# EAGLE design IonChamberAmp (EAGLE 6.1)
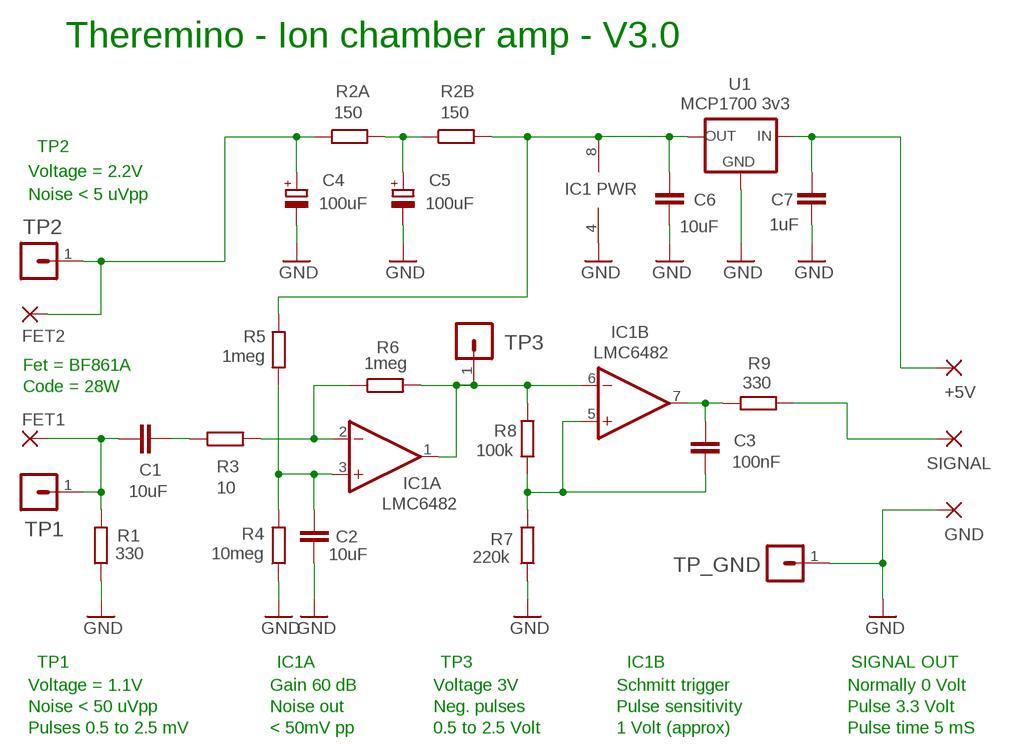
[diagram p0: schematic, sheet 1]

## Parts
+5V  WIREPAD1,6/0,8  [1,6/0,8]
C1  10uF  C-EUC0805  [C0805]
C2  10uF  C-EUC0805  [C0805]
C3  100nF  C-EUC0805  [C0805]
C4  100uF  CPOL-EUE2-5B  [E2-5B]
C5  100uF  CPOL-EUE2-5B  [E2-5B]
C6  10uF  C-EUC0805  [C0805]
C7  1uF  C-EUC0805  [C0805]
FET1  WIREPADSMD1,90-2,54  [SMD1,90-2,54]
FET2  WIREPADSMD1,90-2,54  [SMD1,90-2,54]
GND  WIREPAD1,6/0,8  [1,6/0,8]
IC1  LMC6482  TL072P  [DIL08]
R1  330  R-EU_R0805  [R0805]
R2A  150  R-EU_R0805  [R0805]
R2B  150  R-EU_R0805  [R0805]
R3  10  R-EU_R0805  [R0805]
R4  10meg  R-EU_R0805  [R0805]
R5  1meg  R-EU_R1206_L  [R1206_L]
R6  1meg  R-EU_R0805  [R0805]
R7  220k  R-EU_R0805  [R0805]
R8  100k  R-EU_R0805  [R0805]
R9  330  R-EU_R0805  [R0805]
SIGNAL  WIREPAD1,6/0,8  [1,6/0,8]
TP1  MA01-1  [MA01-1]
TP2  MA01-1  [MA01-1]
TP3  MA01-1  [MA01-1]
TP_GND  MA01-1  [MA01-1]
U1  MCP1700 3v3  MCP1700SOT23L  [SOT23_L]

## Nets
GND: C2.1 C4.- C5.- C6.2 C7.2 GND.1(P) IC1.4(P:V-) R1.1 R4.1 R7.1 TP_GND.1 U1.1(GND)
N$1: C3.2 IC1.5(B:+IN) R7.2 R8.1
N$2: C2.2 IC1.3(A:+IN) R4.2 R5.1
N$3: IC1.1(A:OUT) IC1.6(B:-IN) R6.2 R8.2 TP3.1
N$4: IC1.2(A:-IN) R3.2 R6.1
N$5: C3.1 IC1.7(B:OUT) R9.1
N$6: C1.2 FET1.1(P) R1.2 TP1.1
N$7: R9.2 SIGNAL.1(P)
N$8: +5V.1(P) C7.1 U1.3(IN)
N$10: C6.1 IC1.8(P:V+) R2B.2 R5.2 U1.2(OUT)
N$11: C1.1 R3.1
N$12: C5.+ R2A.2 R2B.1
TP2: C4.+ FET2.1(P) R2A.1 TP2.1

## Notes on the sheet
- Theremino - Ion chamber amp - V3.0
- TP2
- Voltage = 2.2V
- IC1 PWR
- Noise < 5 uVpp
- Fet = BF861A
- Code = 28W
- TP1 | IC1A | TP3 | IC1B | SIGNAL OUT
- Voltage = 1.1V | Gain 60 dB | Voltage 3V | Schmitt trigger | Normally 0 Volt
- Noise < 50 uVpp | Noise out | Neg. pulses | Pulse sensitivity | Pulse 3.3 Volt
- Pulses 0.5 to 2.5 mV | < 50mV pp | 0.5 to 2.5 Volt | 1 Volt (approx) | Pulse time 5 mS

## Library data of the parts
+5V FET1 FET2 GND SIGNAL = 00-LIVIO:WIREPAD: Wire PAD connect wire on PCB
C1-C3 C6 C7 = 00-LIVIO:C-EU: CAPACITOR, European symbol
C4 C5 = 00-LIVIO:CPOL-EU: POLARIZED CAPACITOR, European symbol
IC1 = linear:TL072: OP AMP
R1 R2A R2B R3-R9 = 00-LIVIO:R-EU_: RESISTOR, European symbol
TP1-TP3 TP_GND = 03-con-lstb-M:MA01-1: PIN HEADER
U1 = 00-LIVIO:MCP1700: Linear regulator Quescient courrent 1.8uA Input 2.3v to 6v Output 1.2v 1.8v 2.5v 3.0v 3.3v 5.0v

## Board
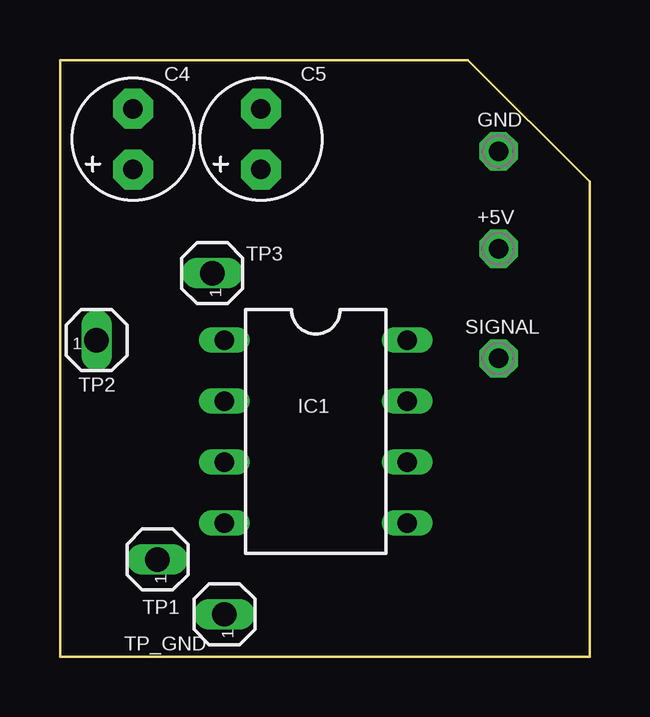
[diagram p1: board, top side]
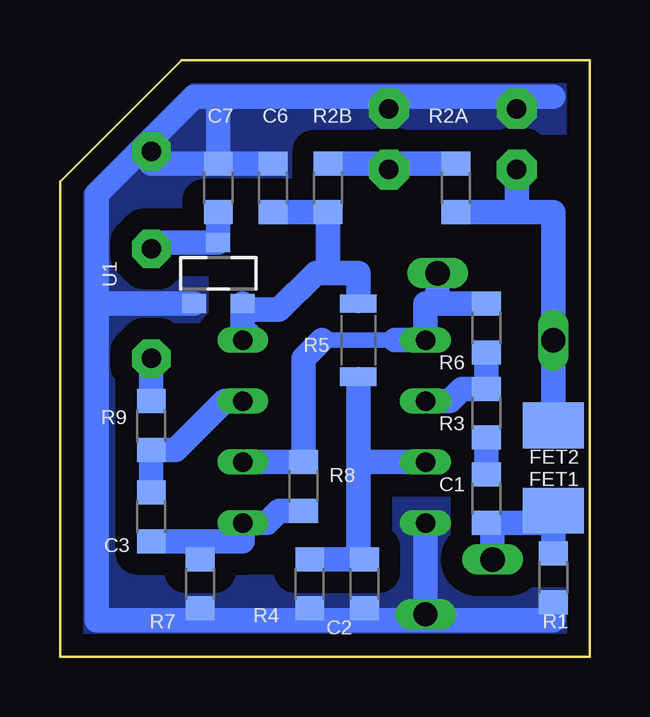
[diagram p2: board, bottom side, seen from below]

Size 22.1 x 24.89 mm. Coordinates in mm from the lower left corner, seen from the top.
Outline: 0,0 22.1,0 22.1,19.81 17.02,24.89 0,24.89 0,0
Copper layers (1*16): Top 0.035mm / dielectric 1.5mm / Bottom 0.035mm
Design rules: minimum track width 10mil, minimum drill 31mil, track to track 31mil, track to pad 31mil, pad to pad 31mil, via to via 31mil, smd to smd 31mil, copper to edge 31mil, drill to drill 8mil, minimum pad ring 5mil, minimum via ring 8mil, stop-mask expansion 4mil, vias tented up to drill 0mil, thermal gap 47mil

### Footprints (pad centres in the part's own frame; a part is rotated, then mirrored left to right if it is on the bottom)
1,6/0,8 = drill 0.813 pad 1.6 octagon: 1 0,0
C0805 = smd 1 x 1.2: 1 -1.016,0; 2 1.016,0
E2-5B = drill 0.813 pad 1.676 octagon: + -1.27,0; - 1.27,0
SMD1,90-2,54 = smd 1.905 x 2.54: 1 0,0
DIL08 = drill 0.813 long: 1 -3.81,-3.81; 2 -1.27,-3.81; 3 1.27,-3.81; 4 3.81,-3.81; 5 3.81,3.81; 6 1.27,3.81; 7 -1.27,3.81; 8 -3.81,3.81
R0805 = smd 1 x 1.2: 1 -1.016,0; 2 1.016,0
R1206_L = smd 0.762 x 1.524: 1 -1.524,0; 2 1.524,0
MA01-1 = drill 1.016 long: 1 0,0
SOT23_L = smd 1 x 0.8: 1 -1.016,-1.27; 2 1.016,-1.27; 3 0,1.27

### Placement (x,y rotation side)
+5V  18.29,17.02 0 top
C1  4.32,6.6 270 bottom
C2  9.4,3.05 90 bottom
C3  18.29,5.84 270 bottom
C4  3.05,21.59 90 top
C5  8.38,21.59 90 top
C6  13.21,19.56 90 bottom
C7  15.49,19.56 90 bottom
FET1  1.52,6.1 90 bottom
FET2  1.52,9.65 270 bottom
GND  18.29,21.08 0 top
IC1  10.67,9.4 270 top
R1  1.52,3.3 90 bottom
R2A  5.59,19.56 90 bottom
R2B  10.92,19.56 270 bottom
R3  4.32,10.16 90 bottom
R4  11.68,3.05 90 bottom
R5  9.65,13.21 90 bottom
R6  4.32,13.72 90 bottom
R7  16.26,3.05 90 bottom
R8  11.94,7.11 90 bottom
R9  18.29,9.65 90 bottom
SIGNAL  18.29,12.45 0 top
TP1  4.06,4.06 90 top
TP2  1.52,13.21 0 top
TP3  6.35,16 90 top
TP_GND  6.86,1.78 90 top
U1  15.49,16 0 bottom

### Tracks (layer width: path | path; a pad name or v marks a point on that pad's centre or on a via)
GND
  Bottom 1.016: 6.86,1.52 1.52,1.52 R1.1 | 6.86,1.52 9.4,1.52 | 9.4,1.52 11.68,1.52 | 11.68,1.52 R4.1 11.68,1.52 | 11.68,1.52 9.4,1.52 | 9.4,1.52 6.86,1.52 | 6.86,1.52 IC1.4 6.86,1.52 | 20.57,14.73 20.57,1.52 | 11.68,1.52 16.26,1.52 | 16.26,1.52 20.57,1.52 | 20.57,14.73 20.57,1.52 | 20.57,1.52 20.57,14.73 | 20.57,14.73 20.57,1.52 | 11.68,1.52 9.4,1.52 | 9.4,1.52 6.86,1.52 | 8.38,23.37 3.56,23.37 | 3.56,23.37 1.52,23.37 | C2.1 9.4,1.52 | U1.1 17.02,14.73 20.57,14.73 | C6.2 C7.2 | R7.1 16.26,1.52 | 3.56,23.37 C4.- | C5.- 8.38,23.37 | 8.38,23.37 15.49,23.37 | 15.49,23.37 16.51,23.37 20.57,19.3 20.57,14.73 | C7.2 15.49,23.37 | GND.1 18.29,20.57 C7.2
  pour Bottom (isolate 0.9, rank 6, no thermals): -1,-1 23.1,-1 23.1,25.89 -1,25.89
N$1
  Bottom 1.016: R8.1 12.95,6.1 13.46,5.59 IC1.5 14.48,4.83 16.26,4.83 | 16.26,4.83 R7.2 16.26,4.83 | 16.26,4.83 C3.2
N$2
  Bottom 0.813: 9.65,11.43 R5.1
  Bottom 1.016: R4.2 9.65,4.06 | 9.65,4.06 C2.2 9.65,4.06 | 9.65,4.06 9.65,8.13 | IC1.3 9.65,8.13 | 9.65,8.13 9.65,11.43
N$3
  Bottom 0.65: 8.13,13.21 11.18,13.21
  Bottom 1.016: 6.35,14.73 6.86,14.73 IC1.1 8.13,13.21 | 6.35,14.73 R6.2 | 11.18,13.21 11.94,12.45 R8.2 | R8.2 13.46,8.13 | 13.46,8.13 IC1.6 13.46,8.13 | 13.46,8.13 R8.2 | 6.35,14.73 TP3.1
N$4
  Bottom 1.016: IC1.2 5.84,10.67 5.33,11.18 R3.2 R6.1
N$5
  Bottom 1.016: C3.1 R9.1 17.27,8.64 15.24,10.67 IC1.7
N$6
  Bottom 1.016: 1.52,5.59 4.06,5.59 | 4.06,5.59 C1.2 | 1.52,5.59 FET1.1 | R1.2 1.52,5.59 | TP1.1 4.06,5.59
N$7
  Bottom 1.016: SIGNAL.1 R9.2
N$8
  Bottom 1.016: +5V.1 18.03,17.27 U1.3 C7.1
N$10
  Bottom 0.813: 9.65,15.24 R5.2
  Bottom 1.016: IC1.8 14.22,13.46 | 9.65,15.24 9.65,16 10.92,16 | IC1.8 14.48,13.46 14.48,14.48 | 14.48,14.48 U1.2 | 10.92,16 11.43,16 12.95,14.48 | 12.95,14.48 14.48,14.48 | 14.48,14.48 IC1.8 | IC1.8 14.48,14.48 | 14.48,14.48 12.95,14.48 | C6.1 R2B.2 10.92,16
N$11
  Bottom 1.016: C1.1 R3.1
N$12
  Bottom 1.016: R2A.2 8.64,20.57 | 8.64,20.57 R2B.1 8.64,20.57 | C5.+ 8.64,20.57
TP2
  Bottom 1.016: 3.05,18.54 1.52,18.54 TP2.1 FET2.1 1.78,9.91 | 3.05,18.54 R2A.1 | C4.+ 3.05,18.54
